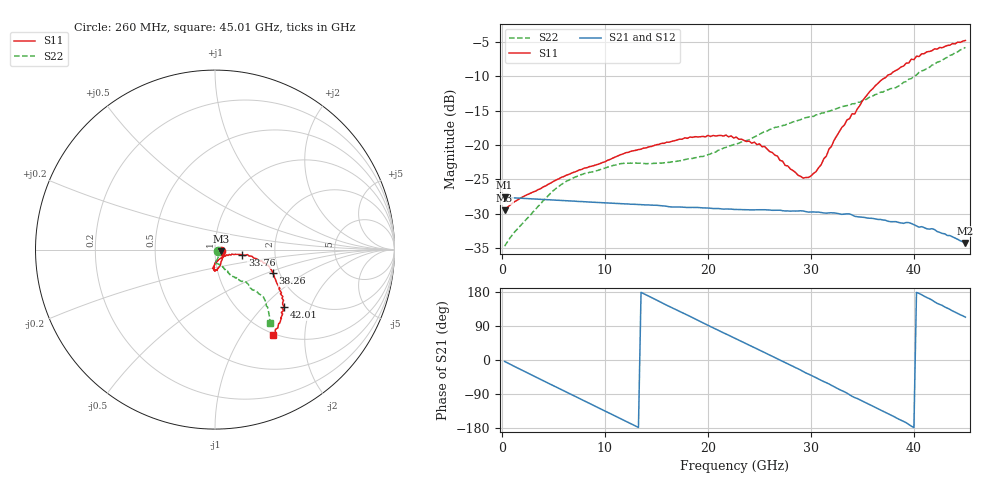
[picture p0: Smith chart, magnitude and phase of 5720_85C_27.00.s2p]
! Device:  ADRF5720
! Description: 0.5dB LSB GaAs MMIC 6-bit Digital Attenuator
! Frequency:  0.000009 -  40 GHz
! Ports:
!	RF1	= Port 1
!	RF2	= Port 2
! Vdd:  3.3 Volt
! Vss:  -3.3 Volt
! Control:  0/3.3 Volt
! State:  27.00 dB attenuation
! Data:  The device was measured using G-S-G Probes on a matrix board.
!  Data was collected using an calibrated 4 port network analyzer.
!  The reference plane for this measurement is at the launchers.
! Note:  Analog Devices supplies this data as a sample of measured data
!  for this product.  Your particular data for this product may vary.
!  Data was taken at 85 degrees C.
!  Analog Devices reserves the right to change this data at anytime.
# GHZ S DB R 45.0
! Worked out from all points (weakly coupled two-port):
!   180 points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, 260 MHz to 45.01 GHz, reference 45 ohm
!   highest |S21| = -27.62 dB at 260 MHz (marker M1); lowest = -34.3 dB at 45.01 GHz (marker M2)
!   lowest |S11| = -29.5 dB at 260 MHz (marker M3), VSWR 1.07, Z = 48 - j0.786 ohm
!   |S11| at or under -10 dB: start of sweep to 37.39 GHz
!   |S22| runs from -34.7 to -5.8 dB; largest |S21 - S12| = 0.00025
!   S11 on the Smith chart (normalised r, x): 260 MHz: 1.07, -0.02; 33.76 GHz: 1.36, -0.09; 38.26 GHz: 1.84, -0.55; 42.01 GHz: 1.56, -1.33; 45.01 GHz: 0.97, -1.38
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0.26  -29.53 -14.2  -27.62 -3.7  -27.62 -3.7  -34.73 -26.4
1.76  -27.77 -6.8  -27.74 -24.4  -27.73 -24.3  -31.81 -20.6
4.76  -25.52 -36.0  -27.99 -64.7  -27.97 -64.6  -26.97 -65.5
6.26  -24.40 -45.2  -28.11 -84.6  -28.10 -84.6  -25.29 -75.0
7.76  -23.56 -52.6  -28.24 -104.6  -28.23 -104.5  -24.30 -81.6
11.51  -21.43 -68.2  -28.55 -154.5  -28.54 -154.4  -22.73 -92.2
15.26  -19.91 -77.7  -28.82 154.7  -28.81 154.9  -22.64 -90.0
18.26  -18.85 -84.5  -29.09 115.2  -29.07 115.4  -21.98 -81.7
22.76  -18.86 -92.2  -29.39 55.5  -29.37 55.7  -19.86 -67.6
25.51  -20.24 -93.0  -29.43 19.6  -29.42 19.8  -18.05 -63.7
29.26  -24.83 -59.4  -29.61 -30.6  -29.59 -30.3  -16.16 -59.4
30.26  -24.14 -40.8  -29.75 -43.4  -29.73 -43.2  -15.85 -58.8
31.01  -22.86 -23.7  -29.84 -53.8  -29.82 -53.5  -15.38 -57.7
33.01  -17.45 -11.2  -30.10 -80.7  -30.08 -80.4  -14.43 -54.9
33.76  -16.16 -11.4  -30.03 -91.8  -30.02 -91.5  -14.22 -53.1
35.76  -12.16 -13.2  -30.67 -118.2  -30.66 -118.1  -12.99 -51.0
37.76  -9.70 -19.0  -31.17 -145.2  -31.15 -145.0  -11.80 -46.3
38.26  -9.17 -22.4  -31.16 -152.2  -31.14 -151.8  -11.66 -46.2
40.26  -7.08 -33.1  -31.79 178.2  -31.76 178.7  -9.83 -45.7
42.01  -6.02 -39.6  -32.31 153.6  -32.31 153.9  -8.27 -44.9
43.51  -5.49 -45.9  -33.19 133.5  -33.15 133.8  -6.97 -48.7
45.01  -4.80 -56.2  -34.27 113.0  -34.24 113.3  -5.82 -53.3
